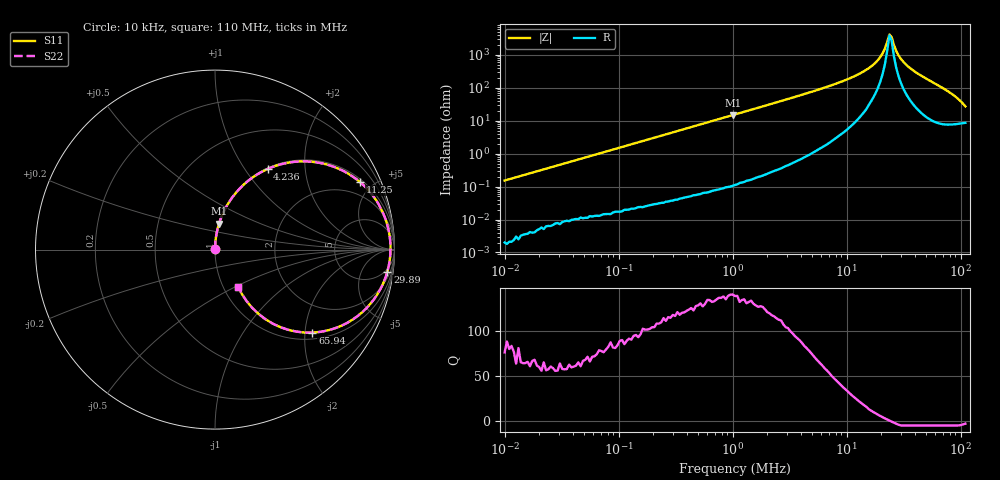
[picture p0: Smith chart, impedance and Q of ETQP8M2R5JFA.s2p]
! *** S-Parameter ***
!Copyright (C)  Panasonic Industry Corporation
!Power Inductors for Automotive application
!Parts No. ETQP8M2R5JFA
# HZ S RI R 50.000000
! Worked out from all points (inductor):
!   201 points, 10 kHz to 110 MHz, reference 50 ohm
!   read as one part in series: L = 2.42 uH near 10.48 kHz
!   highest Q = 138 at 1.001 MHz (marker M1), where L = 2.34 uH
!   self-resonance near 23.69 MHz
!   S11 on the Smith chart (normalised r, x): 10 kHz: 1.00, +0.00; 4.236 MHz: 1.02, +1.28; 11.25 MHz: 1.15, +4.20; 29.89 MHz: 4, -15; 65.94 MHz: 1.16, -2.19; 110 MHz: 1.17, -0.52
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10000  2.24e-05 0.00153  1 -0.00153  1 -0.00153  2.24e-05 0.00153
48644.84  0.000163 0.00729  0.9998 -0.00729  0.9998 -0.00729  0.000163 0.00729
225874.2  0.00143 0.0334  0.9986 -0.0334  0.9986 -0.0334  0.00143 0.0334
1001128  0.0223 0.1441  0.9777 -0.1441  0.9777 -0.1441  0.0223 0.1441
1048809  0.0244 0.1506  0.9756 -0.1506  0.9756 -0.1506  0.0244 0.1506
2313208  0.1072 0.305  0.8928 -0.305  0.8928 -0.305  0.1072 0.305
4235506  0.2931 0.4492  0.7069 -0.4492  0.7069 -0.4492  0.2931 0.4492
5101914  0.3813 0.4788  0.6187 -0.4788  0.6187 -0.4788  0.3813 0.4788
7755250  0.6134 0.4765  0.3866 -0.4765  0.3866 -0.4765  0.6134 0.4765
1.125256e7  0.8071 0.377  0.1929 -0.377  0.1929 -0.377  0.8071 0.377
1.558476e7  0.9224 0.2321  0.0776 -0.2321  0.0776 -0.2321  0.9224 0.2321
1.877276e7  0.9606 0.1357  0.0394 -0.1357  0.0394 -0.1357  0.9606 0.1357
2.158485e7  0.975 0.06  0.025 -0.06  0.025 -0.06  0.975 0.06
2.368988e7  0.978 0.00853  0.022 -0.00853  0.022 -0.00853  0.978 0.00853
2.481818e7  0.9774 -0.0175  0.0226 0.0175  0.0226 0.0175  0.9774 -0.0175
2.723854e7  0.9719 -0.0697  0.0281 0.0697  0.0281 0.0697  0.9719 -0.0697
2.989494e7  0.9605 -0.122  0.0395 0.122  0.0395 0.122  0.9605 -0.122
3.437309e7  0.9314 -0.2003  0.0686 0.2003  0.0686 0.2003  0.9314 -0.2003
4.14044e7  0.8666 -0.3012  0.1334 0.3012  0.1334 0.3012  0.8666 -0.3012
6.593501e7  0.5431 -0.4624  0.4569 0.4624  0.4569 0.4624  0.5431 -0.4624
8.716816e7  0.28 -0.3871  0.72 0.3871  0.72 0.3871  0.28 -0.3871
1.1e8  0.1287 -0.2073  0.8713 0.2073  0.8713 0.2073  0.1287 -0.2073
